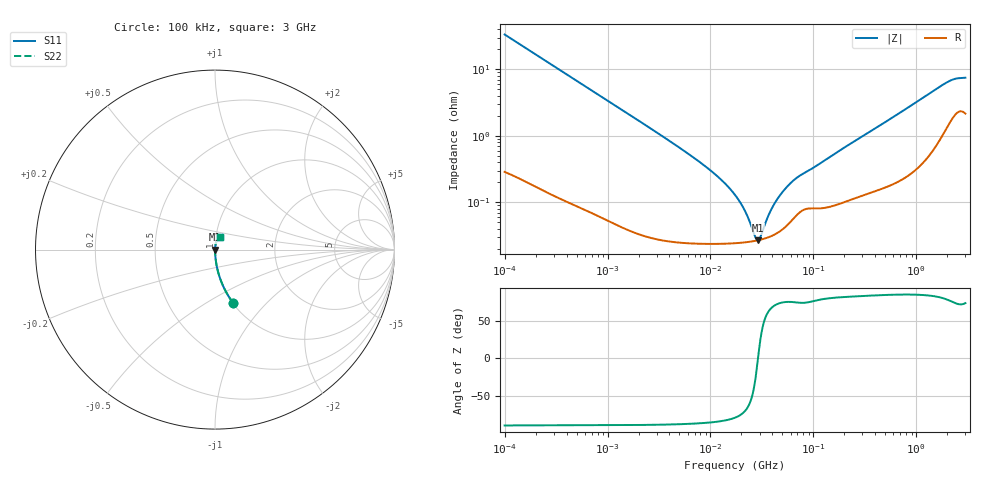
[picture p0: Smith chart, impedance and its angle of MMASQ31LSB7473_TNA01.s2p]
! MMASQ31LSB7473_TNA01  S-PARAMETER MODEL  ( Standard Model )
! Model Generated by TAIYO YUDEN Corporation (http://www.ty-top.com)
! Version 1.0
! TAIYO YUDEN Control No. 220601
! Copyright(c) 2013 TAIYO YUDEN CO.,LTD. All Rights Reserved.
! Product Description (link to TY-COMPAS)
! https://ds.yuden.co.jp/TYCOMPAS/or/detail?pn=MMASQ31LSB7473KTNA01&u=M
! Products Name : Multilayer Ceramic Capacitors
! Characteristics :
!  Capacitance : 0.047 [uF] , Rated Voltage : 250 [V] , TCC : X7R
!  Case Size : 3.2 x 1.6 / 0.126 x 0.063 [mm/inch] , Thickness : 1.6 / 0.063 [mm/inch]
!  (Conditions: Temperature = 25 [degC] , DC Bias Voltage = 0 [V])
! External Node Assignments :
!  1  o---| |---o  2
! GND o---------o GND
! Frequency Range : 100kHz  -  3GHz  [ 401 STEP ]
# MHZ S RI R 50
! Freq[MHz].  S11 Real  S11 Imag  S21 Real  S21 Imag  S12 Real  S12 Imag  S22 Real  S22 Imag
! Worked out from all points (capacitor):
!   401 points, 100 kHz to 3 GHz, reference 50 ohm
!   read as one part in series: C = 47.6 nF near 105.3 kHz
!   lowest |Z| = 26.8 mohm at 29 MHz (marker M1)
!   series resonance near 28.99 MHz, so ESL is about 630 pH
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0.1  0.1023 -0.2988  0.8977 0.2988  0.8977 0.2988  0.1023 -0.2988
0.228123  0.0226 -0.1435  0.9774 0.1435  0.9774 0.1435  0.0226 -0.1435
0.562235  0.00439 -0.0597  0.9956 0.0597  0.9956 0.0597  0.00439 -0.0597
3.161081  0.000387 -0.0107  0.9996 0.0107  0.9996 0.0107  0.000387 -0.0107
6.178009  0.000269 -0.00527  0.9997 0.00527  0.9997 0.00527  0.000269 -0.00527
9.824692  0.000246 -0.00308  0.9998 0.00308  0.9998 0.00308  0.000246 -0.00308
13.7349  0.000242 -0.00193  0.9998 0.00193  0.9998 0.00193  0.000242 -0.00193
17.7727  0.000244 -0.0012  0.9998 0.0012  0.9998 0.0012  0.000244 -0.0012
21.84217  0.00025 -0.000677  0.9997 0.000677  0.9997 0.000677  0.00025 -0.000677
27.54426  0.000264 -0.000121  0.9997 0.000121  0.9997 0.000121  0.000264 -0.000121
29.00125  0.000268 1.27e-06  0.9997 -1.27e-06  0.9997 -1.27e-06  0.000268 1.27e-06
30.53531  0.000273 0.000124  0.9997 -0.000124  0.9997 -0.000124  0.000273 0.000124
35.64176  0.000293 0.000495  0.9997 -0.000495  0.9997 -0.000495  0.000293 0.000495
39.51212  0.000313 0.000749  0.9997 -0.000749  0.9997 -0.000749  0.000313 0.000749
48.55934  0.000378 0.00129  0.9996 -0.00129  0.9996 -0.00129  0.000378 0.00129
56.67997  0.000466 0.00171  0.9995 -0.00171  0.9995 -0.00171  0.000466 0.00171
66.15861  0.000603 0.00214  0.9994 -0.00214  0.9994 -0.00214  0.000603 0.00214
97.38194  0.000818 0.00312  0.9992 -0.00312  0.9992 -0.00312  0.000818 0.00312
547.5153  0.00207 0.0174  0.9979 -0.0174  0.9979 -0.0174  0.00207 0.0174
1935.725  0.0158 0.0594  0.9842 -0.0594  0.9842 -0.0594  0.0158 0.0594
2378.954  0.0246 0.0658  0.9754 -0.0658  0.9754 -0.0658  0.0246 0.0658
3000  0.0259 0.0682  0.9741 -0.0682  0.9741 -0.0682  0.0259 0.0682
